FUNCTION_BLOCK FB_LN_IED_LD1_XCBR1 EXTENDS FB_AcsiCommonLogicalNodeClass
VAR_INPUT
	Beh: FB_DO_IED_LD1_XCBR1_Beh := (sClass:='ENS', bLinkResult:=THIS^.AddDataToContainer(ipData:=Beh));
	Loc: FB_DO_IED_LD1_XCBR1_Loc := (sClass:='SPS', bLinkResult:=THIS^.AddDataToContainer(ipData:=Loc));
	OpCnt: FB_DO_IED_LD1_XCBR1_OpCnt := (sClass:='INS', bLinkResult:=THIS^.AddDataToContainer(ipData:=OpCnt));
	Pos: FB_DO_IED_LD1_XCBR1_Pos := (sClass:='DPC', bLinkResult:=THIS^.AddDataToContainer(ipData:=Pos));
	BlkOpn: FB_DO_IED_LD1_XCBR1_BlkOpn := (sClass:='SPC', bLinkResult:=THIS^.AddDataToContainer(ipData:=BlkOpn));
	BlkCls: FB_DO_IED_LD1_XCBR1_BlkCls := (sClass:='SPC', bLinkResult:=THIS^.AddDataToContainer(ipData:=BlkCls));
END_VAR
VAR
END_VAR

END_FUNCTION_BLOCK
